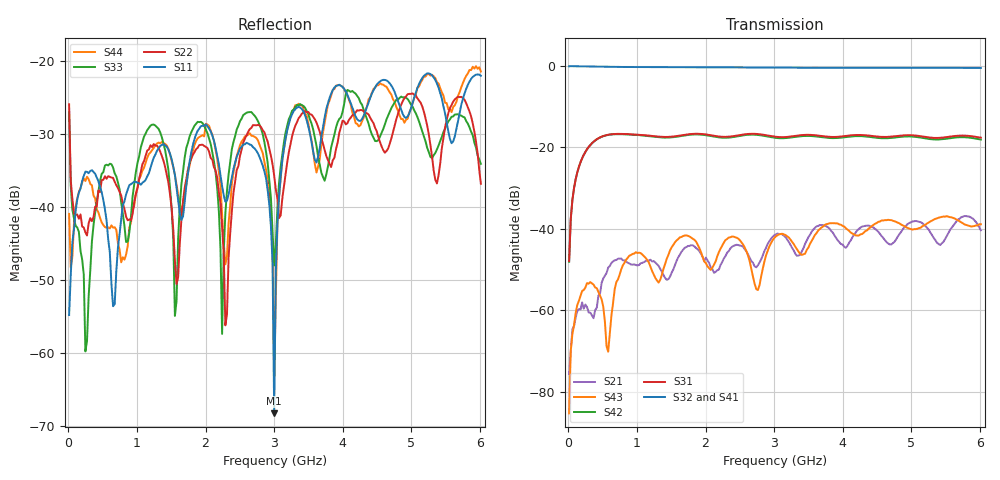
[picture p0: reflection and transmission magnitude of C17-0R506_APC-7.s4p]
! MARKI MICROWAVE INC.
! Email:  support@markimicrowave.com  Phone:  408-778-4200
! Model Number:  C17-0R506  Date:  04/16
! Filename:		C17_0R506_APC-7.S4P  Version: 1.0
! Description:  4-port S-parameter data for Directional Coupler C17-0R506 with APC-7 connectors on the through ports and SMA on
!  the coupled ports
! Frequency Range: 	10 MHz to 6 GHz
! Port Configuration:	PORT 1: Input
!  PORT 2: Isolated
!  Port 3: Coupled
!  Port 4: Output
! S4P File: Measurements: Mag<S11> Ang<S11> Mag<S12> Ang<S12> Mag<S13> Ang<S13> Mag<S14> Ang<S14>! row 1
!  Mag<S21> Ang<S21> Mag<S22> Ang<S22> Mag<S23> Ang<S23> Mag<S24> Ang<S24>! row 2
!  Mag<S31> Ang<S31> Mag<S32> Ang<S32> Mag<S33> Ang<S33> Mag<S34> Ang<S34>! row 3
!  Mag<S41> Ang<S41> Mag<S42> Ang<S42> Mag<S43> Ang<S43> Mag<S44> Ang<S44>! row 4
# Hz S  dB  R 50
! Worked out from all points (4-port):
!   254 points, 10 MHz to 6.016 GHz, reference 50 ohm
!   strongest paths, dB at 10 MHz, 1.505 GHz, 3.025 GHz, 4.52 GHz, 6.016 GHz:
!     S32: -0.1, -0.3, -0.4, -0.4, -0.5
!     S41: 0.0, -0.3, -0.4, -0.5, -0.5
!     S31: -47.9, -17.3, -17.4, -17.3, -17.6
!     S42: -48.1, -17.5, -17.7, -17.7, -18.0
!     S43: -85.3, -44.5, -41.8, -38.3, -38.8
!     S21: -75.6, -50.8, -41.4, -40.7, -40.3
!   lowest |S11| = -68.3 dB at 3.001 GHz (marker M1), VSWR 1.00, Z = 50 + j0.00716 ohm
!   |S11| at or under -10 dB: start of sweep to end of sweep
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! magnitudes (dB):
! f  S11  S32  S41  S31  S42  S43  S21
! 10 MHz  -54.8  -0.1  0.0  -47.9  -48.1  -85.3  -75.6
! 247.4 MHz  -35.1  -0.1  -0.1  -21.1  -21.1  -54.4  -58.6
! 2.289 GHz  -39.3  -0.3  -0.3  -17.4  -17.6  -42.8  -46.7
! 2.669 GHz  -31.5  -0.4  -0.4  -16.6  -16.8  -49.9  -47.9
! 3.001 GHz  -68.3  -0.4  -0.4  -17.3  -17.6  -42.3  -41.6
! 3.286 GHz  -26.8  -0.4  -0.4  -17.2  -17.5  -43.7  -45.3
! 6.016 GHz  -22.0  -0.5  -0.5  -17.6  -18.0  -38.8  -40.3
